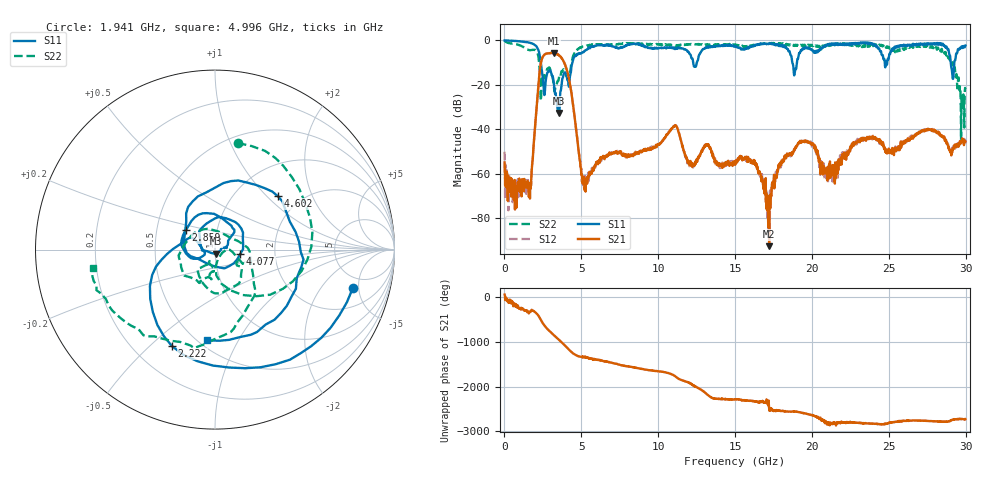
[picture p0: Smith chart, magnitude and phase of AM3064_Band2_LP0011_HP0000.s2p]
# Hz S DB R 50.0
!freq dBS11 angS11 dBS21 angS21 dBS12 angS12 dBS22 angS22
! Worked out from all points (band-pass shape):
!   1600 points, 10 MHz to 29.98 GHz, reference 50 ohm
!   highest |S21| = -5.61 dB at 3.234 GHz (marker M1); lowest = -92.6 dB at 17.22 GHz (marker M2)
!   |S21| within 3 dB of the highest: 2.424 GHz to 3.783 GHz (1.359 GHz wide, 43.8 % of centre)
!   lowest |S11| = -32.7 dB at 3.553 GHz (marker M3), VSWR 1.05, Z = 50.3 - j2.3 ohm
!   |S11| at or under -10 dB: 2.365 GHz to 4.423 GHz (2.057 GHz wide, 60.6 % of centre); 18.73 GHz to 19.02 GHz (294.6 MHz wide, 1.56 % of centre); 29.03 GHz to 29.26 GHz (229.4 MHz wide, 0.787 % of centre)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
!   |S22| runs from -45.0 to -0.2 dB; largest |S21 - S12| = 0.014
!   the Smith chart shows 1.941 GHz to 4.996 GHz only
!   S11 on the Smith chart (normalised r, x): 1.941 GHz: 3.67, -4.30; 2.222 GHz: 0.36, -0.59; 2.859 GHz: 0.71, +0.16; 4.077 GHz: 1.33, -0.07; 4.602 GHz: 1.53, +1.16; 4.996 GHz: 0.55, -0.75
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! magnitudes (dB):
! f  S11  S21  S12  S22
! 10 MHz  0.0  -54.9  -50.1  -0.2
! 1.566 GHz  -1.0  -65.8  -67.9  -4.3
! 1.941 GHz  -2.0  -43.4  -43.1  -4.3
! 2.222 GHz  -4.6  -19.2  -19.0  -8.0
! 2.859 GHz  -14.2  -5.8  -5.8  -12.5
! 3.234 GHz  -21.1  -5.6  -5.7  -22.1
! 3.553 GHz  -32.7  -6.8  -6.6  -16.4
! 4.077 GHz  -16.9  -13.7  -13.7  -17.1
! 4.602 GHz  -6.8  -36.7  -36.5  -5.0
! 4.996 GHz  -5.9  -59.9  -57.5  -3.2
! 5.015 GHz  -5.8  -60.6  -59.9  -3.2
! 10 GHz  -3.5  -46.8  -46.9  -1.8
! 15 GHz  -2.5  -56.0  -54.9  -1.9
! 16.32 GHz  -2.2  -55.0  -55.2  -2.0
! 17.22 GHz  -1.4  -92.6  -76.7  -1.5
! 18.17 GHz  -2.6  -54.5  -52.9  -2.1
! 19.99 GHz  -4.1  -46.8  -46.6  -2.0
! 20.93 GHz  -2.2  -60.0  -58.9  -2.1
! 25 GHz  -7.9  -48.7  -49.9  -2.9
! 28.56 GHz  -2.2  -43.6  -43.6  -4.6
! 29.18 GHz  -17.4  -49.2  -48.3  -10.3
! 29.98 GHz  -2.3  -45.5  -46.6  -21.8
